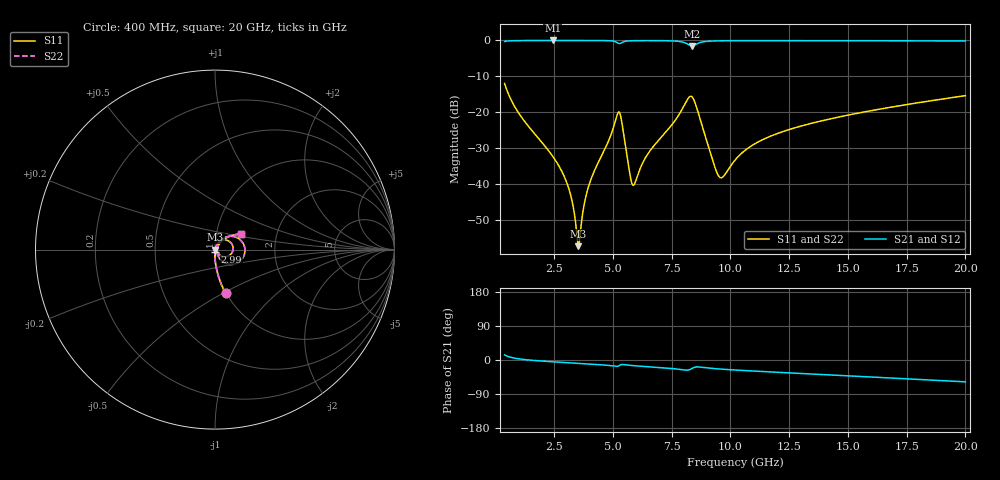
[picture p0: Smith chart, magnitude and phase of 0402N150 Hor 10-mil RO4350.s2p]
# MHz S  dB  R 50
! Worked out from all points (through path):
!   1961 points, 400 MHz to 20 GHz, reference 50 ohm
!   highest |S21| = -0.01 dB at 2.45 GHz (marker M1); lowest = -1.5 dB at 8.37 GHz (marker M2)
!   group delay of S21, straight-line fit = 8.38 ps
!   lowest |S11| = -57.2 dB at 3.54 GHz (marker M3), VSWR 1.00, Z = 50.1 - j0.0337 ohm
!   |S11| at or under -10 dB: start of sweep to end of sweep
!   |S22| runs from -57.2 to -12.0 dB; largest |S21 - S12| = 0
!   S11 on the Smith chart (normalised r, x): 400 MHz: 0.99, -0.52; 2.99 GHz: 1.00, -0.02; 20 GHz: 1.32, +0.24
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400  -11.99 -76.3  -0.29 13.6  -0.29 13.6  -11.99 -76.3
1040  -20.61 -86.8  -0.04 2.7  -0.04 2.7  -20.61 -86.8
2450  -32.26 -92.4  -0.01 -4.7  -0.01 -4.7  -32.26 -92.4
2990  -38.65 -91.2  -0.01 -6.8  -0.01 -6.8  -38.65 -91.2
3260  -44.38 -86.0  -0.01 -7.8  -0.01 -7.8  -44.38 -86.0
3540  -57.22 -14.1  -0.01 -8.8  -0.01 -8.8  -57.22 -14.1
3670  -50.56 51.3  -0.01 -9.3  -0.01 -9.3  -50.56 51.3
3820  -44.45 64.9  -0.01 -9.9  -0.01 -9.9  -44.45 64.9
4020  -39.62 69.4  -0.02 -10.6  -0.02 -10.6  -39.62 69.4
5220  -20.15 19.8  -0.74 -16.4  -0.74 -16.4  -20.15 19.8
5360  -21.82 -26.8  -0.71 -12.2  -0.71 -12.2  -21.82 -26.8
5720  -36.82 -36.8  -0.12 -13.9  -0.12 -13.9  -36.82 -36.8
5860  -40.28 1.3  -0.08 -14.8  -0.08 -14.8  -40.28 1.3
6940  -27.84 61.8  -0.06 -19.6  -0.06 -19.6  -27.84 61.8
8030  -18.16 36.5  -0.57 -26.3  -0.57 -26.3  -18.16 36.5
8370  -15.69 -13.0  -1.54 -22.3  -1.54 -22.3  -15.69 -13.0
9500  -37.68 -23.4  -0.12 -23.5  -0.12 -23.5  -37.68 -23.4
10200  -33.30 43.6  -0.07 -26.4  -0.07 -26.4  -33.30 43.6
11370  -27.62 52.9  -0.05 -30.4  -0.05 -30.4  -27.62 52.9
13470  -23.02 49.9  -0.06 -37.0  -0.06 -37.0  -23.02 49.9
16740  -18.67 41.0  -0.10 -47.2  -0.10 -47.2  -18.67 41.0
20000  -15.36 31.1  -0.17 -57.6  -0.17 -57.6  -15.36 31.1
